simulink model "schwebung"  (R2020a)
settings: Solver=ode45  StartTime=0.0  StopTime=100  MaxStep=0.1  RelTol=1e-3  EnableMultiTasking=on

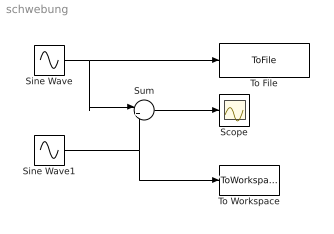
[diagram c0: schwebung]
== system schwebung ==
  Scope : Scope
  Sine Wave : Sin  SampleTime=0
  Sine Wave1 : Sin  Frequency=1.1  SampleTime=0
  Sum : Sum  Inputs=|++
  To File : ToFile  Filename=schwingung1.mat  SaveFormat=Timeseries
  To Workspace : ToWorkspace  VariableName=simout  SaveFormat=Structure  SampleTime=-1
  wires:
  Sine Wave/1 -> Sum/1, To File/1
  Sine Wave1/1 -> Sum/2, To Workspace/1
  Sum/1 -> Scope/1
